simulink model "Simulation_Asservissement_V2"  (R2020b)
settings: Solver=VariableStepAuto  StartTime=0.0  StopTime=12  RelTol=1e-3
libraries: fl_lib x10, nesl_utility x6, ee_lib x1, sdl_lib x1, pid_lib x1

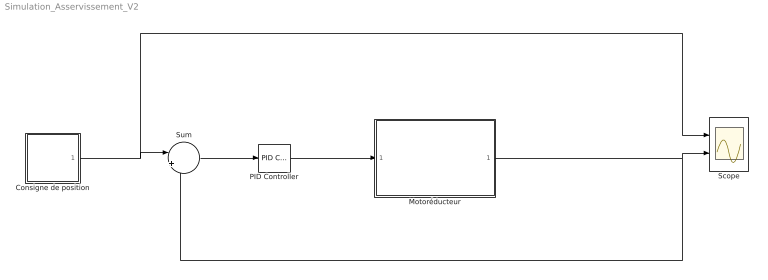
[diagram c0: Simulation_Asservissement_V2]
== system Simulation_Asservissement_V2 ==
  Consigne de position : Subsystem
  Motoréducteur : Subsystem  mask{r_induit=0, k=0.0106, r1=1, Io=0, Rend=100}
      mask prompts: r_induit "Resistance d induit (ohm)"; k "Constante de couple (Nm/A)"; r1 "Rapport de reduction"; Io "Courant a vide (A)"; Rend "Rendement reducteur (%)"
  PID Controller : pid_lib/PID Controller  Controller=PID  Form=Parallel  TimeDomain=Continuous-time  UseExternalTs=off  SampleTime=-1  IntegratorMethod=Forward Euler  FilterMethod=Forward Euler  ControllerParametersSource=internal  P=0.01  I=0  D=0  UseFilter=on  N=150  TunerSelectOption=Transfer Function Based (PID Tuner App)  InitialConditionSource=internal  InitialConditionForIntegrator=0  InitialConditionForFilter=0  DifferentiatorICPrevScaledInput=0  ExternalReset=none  TrackingMode=off  Kt=1  LimitOutput=off  SatLimitsSource=internal  UpperSaturationLimit=inf  LowerSaturationLimit=-inf  LinearizeAsGain=on  AntiWindupMode=none  Kb=1  POutMin=[]  POutMax=[]  IOutMin=[]  IOutMax=[]  DOutMin=[]  DOutMax=[]  NOutMin=[]  NOutMax=[]  SumOutMin=[]  SumOutMax=[]  SaturationOutMin=[]  SaturationOutMax=[]  PParamMin=[]  PParamMax=[]  IParamMin=[]  IParamMax=[]  DParamMin=[]  DParamMax=[]  NParamMin=[]  NParamMax=[]  KbParamMin=[]  KbParamMax=[]  KtParamMin=[]  KtParamMax=[]  KbOutMin=[]  KbOutMax=[]  KtOutMin=[]  KtOutMax=[]  IntegratorOutMin=[]  IntegratorOutMax=[]  FilterOutMin=[]  FilterOutMax=[]  SumI1OutMin=[]  SumI1OutMax=[]  SumI2OutMin=[]  SumI2OutMax=[]  SumI3OutMin=[]  SumI3OutMax=[]  SumI4OutMin=[]  SumI4OutMax=[]  SumDOutMin=[]  SumDOutMax=[]  DifferentiatorOutMin=[]  DifferentiatorOutMax=[]  FilterDiffOutCoefMin=[]  FilterDiffOutCoefMax=[]  ReciprocalOutMin=[]  ReciprocalOutMax=[]  SumDenOutMin=[]  SumDenOutMax=[]  SumNumOutMin=[]  SumNumOutMax=[]  DivideOutMin=[]  DivideOutMax=[]  UdiffTsProdOutMin=[]  UdiffTsProdOutMax=[]  NTsProdOutMin=[]  NTsProdOutMax=[]  UintegralTsProdOutMin=[]  UintegralTsProdOutMax=[]  UngainTsProdOutMin=[]  UngainTsProdOutMax=[]  IntegratorContinuousStateAttributes=''  IntegratorStateMustResolveToSignalObject=off  IntegratorRTWStateStorageClass=Auto  FilterContinuousStateAttributes=''  FilterStateMustResolveToSignalObject=off  FilterRTWStateStorageClass=Auto  ParallelPVariant=InternalParameters  IdealPVariant=Disabled  IVariant=InternalParameters  DVariant=InternalParameters  IntegratorVariant=Continuous  SatVariant=Disabled  AWVariant=Passthrough  PCopyVariant=Disabled  TRVariant=Disabled  FdbkBlocksVariant=Forward  IdealPFdbkVariant=Disabled  SatFdbkVariant=Disabled  DerivativeFilterVariant=ContFilter  NVariant=InternalParameters  NCopyVariant=Disabled  FilterICVariant=InternalICsFilter  IntegratorICVariant=InternalICs  ExternalResetVariant=Disabled  TRSumVariant=Passthrough  SumFdbkVariant=Disabled  SumVariant=Sum_PID  TsampFilterVariant=InternalTs  TsampNgainVariant=Passthrough  TsampIntegralVariant=Passthrough  ExternalSaturationOutDataTypeStr=Inherit: Same as second input
  Scope : Scope  NumInputPorts=2
  Sum : Sum  Inputs=|+-
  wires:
  Sum/1 -> PID Controller/1
  Motoréducteur/1(Out1) -> Scope/2, Sum/2
  PID Controller/1 -> Motoréducteur/1(In1)
  Consigne de position/1(Out1) -> Scope/1, Sum/1

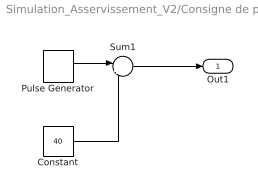
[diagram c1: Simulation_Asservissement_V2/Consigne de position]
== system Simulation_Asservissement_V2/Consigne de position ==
  Constant : Constant  Value=40
  Pulse Generator : DiscretePulseGenerator  PulseType=Time based  Amplitude=40  Period=4  PulseWidth=50
  Sum1 : Sum  Inputs=|++
  Out1 : Outport  VectorParamsAs1DForOutWhenUnconnected=off
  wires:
  Pulse Generator/1 -> Sum1/1
  Sum1/1 -> Out1/1
  Constant/1 -> Sum1/2

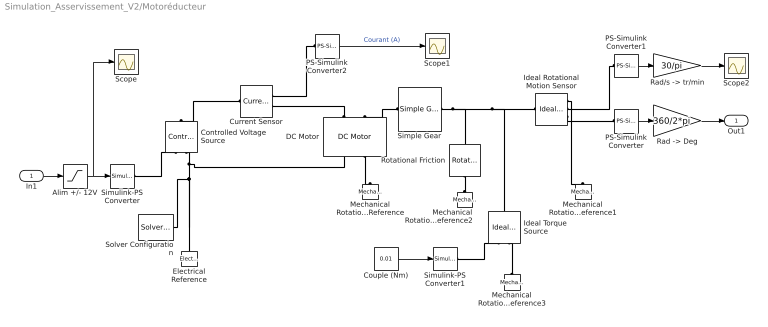
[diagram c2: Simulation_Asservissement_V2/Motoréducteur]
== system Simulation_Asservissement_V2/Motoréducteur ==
  In1 : Inport
  Alim +/- 12V : Saturate  UpperLimit=12  LowerLimit=-12
  Controlled Voltage Source : fl_lib/Electrical/Electrical Sources/Controlled Voltage Source
  Couple (Nm) : Constant  Value=0.01
  Current Sensor : fl_lib/Electrical/Electrical Sensors/Current Sensor
  DC Motor : ee_lib/Electromechanical/Brushed Motors/DC Motor  field_option=ee.enum.field_option.pm  Rf=100 Ohm  Lf=1 H  Laf=0.15 H  If0=0 A  parameterization=1  Ra=r_induit+0.01 Ohm  La=1.2e-2 H  emf_or_torque=2  Kv=k V/(rad/s)  Ki=k N*m/A  T_stall=2.4e-4 N*m  w_max=1.91e+4 rpm  w_rated=1.5e+4 rpm  P_rated=0.08 W  V_rated=1.5 V  J=1e-6 kg*m^2  lam_param=2  lam=0 N*m/(rad/s)  i_noload=Io A  V_i_noload=12 V  speed0=0 rpm  enable_fault_armature=ee.enum.faults.faultEnable.no  rev_faulted=1 / 3  G_faulted_armature=1e-5 S  fault_trigger_armature=ee.enum.faults.faultTrigger.temporal  t_fault_armature=1 s  max_permissible_current_armature=inf A  t_fail_on_current_armature=1 s  enable_fault_field=ee.enum.faults.faultEnable.no  G_faulted_field=1e-5 S  fault_trigger_field=ee.enum.faults.faultTrigger.temporal  t_fault_field=1 s  max_permissible_current_field=inf A  t_fail_on_current_field=1 s  fault_action=ee.enum.faults.faultAction.none  alpha=3.93e-3 1/K  Tmeas=25 degC  thermal_mass=100 J/K  initial_temperature=25 degC
  Electrical Reference : fl_lib/Electrical/Electrical Elements/Electrical Reference
  Ideal Rotational Motion Sensor : fl_lib/Mechanical/Mechanical Sensors/Ideal Rotational Motion Sensor  wrap_angle=simscape.enum.onoff.off  offset=0 rad
  Ideal Torque Source : fl_lib/Mechanical/Mechanical Sources/Ideal Torque Source
  Mechanical Rotational Reference{,1..3} (4 alike) : fl_lib/Mechanical/Rotational Elements/Mechanical Rotational Reference
  PS-Simulink Converter : nesl_utility/PS-Simulink Converter  PhysicalDomain=network_engine_domain  SubClassName=ps_output  LeftPortType=input  RightPortType=output  PseudoPeriodic=off  Frequencies=[]  Unit=1  AffineConversion=off
  PS-Simulink Converter1 : nesl_utility/PS-Simulink Converter  PhysicalDomain=network_engine_domain  SubClassName=ps_output  LeftPortType=input  RightPortType=output  PseudoPeriodic=off  Frequencies=[]  Unit=1  AffineConversion=off
  PS-Simulink Converter2 : nesl_utility/PS-Simulink Converter  PhysicalDomain=network_engine_domain  SubClassName=ps_output  LeftPortType=input  RightPortType=output  PseudoPeriodic=off  Frequencies=[]  Unit=1  AffineConversion=off
  "Rad -> Deg" : Gain  Gain=360/2*pi
  "Rad/s -> tr/min" : Gain  Gain=30/pi
  Rotational Friction : fl_lib/Mechanical/Rotational Elements/Rotational Friction  brkwy_trq=0.01 N*m  brkwy_vel=0.02 rad/s  Col_trq=0.01 N*m  visc_coef=0 N*m/(rad/s)  w_specify=off  w_priority=None  w=0 rad/s  w_nominal_specify=off  w_nominal_unit=rad/s  w_nominal_value=1  t_specify=off  t_priority=None  t=0 N*m  t_nominal_specify=off  t_nominal_unit=N*m  t_nominal_value=1
  Scope : Scope
  Scope1 : Scope
  Scope2 : Scope
  Simple Gear : sdl_lib/Gears/Simple Gear  ratio=1/r1  rotation_direction=3-2*(1)  friction_model=2  mu_visc=[0, 0] N*m/(rad/s)  T_noload=0.1 N*m  T_nom=5 N*m  efficiency_nom=0.8  efficiency=Rend/100  temperature_TLU=[280, 300, 320] K  load_TLU=[1, 5, 10] N*m  efficiency_TLU=[.95, .9, .85]  efficiency_TLU2=[.85, .8, .75; .95, .9, .85; .85, .8, .7]  w_thr=0.01 rad/s  pwr_thr=0.001 W  thermal_mass=50 J/K  enable_faults=simscape.enum.onoff.off  efficiency_fault=0.05  external_fault=simscape.enum.onoff.off  temporal_fault=simscape.enum.onoff.off  fault_time=5 s  fault_angles=pi / 12 rad  report_fault=simscape.enum.assert.action.none  temperature_specify=off  temperature_priority=High  temperature=300 K  temperature_nominal_specify=off  temperature_nominal_unit=K  temperature_nominal_value=1
  Simulink-PS Converter : nesl_utility/Simulink-PS Converter  PhysicalDomain=network_engine_domain  SubClassName=ps_input  LeftPortType=input  RightPortType=output  PseudoPeriodic=off  Frequencies=[]  NoiseDistribution=none  NoiseParameters=[]  Unit=1  AffineConversion=off  FilteringAndDerivatives=provide  SimscapeFilterOrder=1  InputFilterTimeConstant=0.001  UdotUserProvided=0
  Simulink-PS Converter1 : nesl_utility/Simulink-PS Converter  PhysicalDomain=network_engine_domain  SubClassName=ps_input  LeftPortType=input  RightPortType=output  PseudoPeriodic=off  Frequencies=[]  NoiseDistribution=none  NoiseParameters=[]  Unit=1  AffineConversion=off  FilteringAndDerivatives=provide  SimscapeFilterOrder=1  InputFilterTimeConstant=0.001  UdotUserProvided=0
  Solver Configuration : nesl_utility/Solver Configuration  PhysicalDomain=network_engine_domain  SubClassName=solver  LeftPortType=input  RightPortType=generic  Tones=[]  Harmonics=[]  SimulateNoise=off  Profile=off  UseLocalSampling=off  EnableSwitchedLinearOptims=on  FrequencyDomain=off  UseCCode=off  RelTol=0.001  AbsTol=1e-06  MinStep=1e-09  ToWorkspace=off  RevertToSquareIcSolve=off  NumHomotopyIterations=100  PhasorMode=off  PhasorModeNumHarmonics=1  DoDC=off  ResidualTolerance=1e-09  UseLocalSolver=off  LocalSolverChoice=NE_BACKWARD_EULER_ADVANCER  LocalSolverSampleTime=0.001  DoFixedCost=off  MaxNonlinIter=3  MaxModeIter=2  ComputeImpulses=off  ImpulseIterations=2  LinearAlgebra=Sparse  EquationFormulation=NE_TIME_EF  DelaysMemoryBudget=1024  AutomaticFiltering=on  FilteringTimeConstant=0.001  PartitionStorageMethod=AS_NEEDED  PartitionMemoryBudget=1024  PartitionMethod=FAST
  Out1 : Outport  VectorParamsAs1DForOutWhenUnconnected=off
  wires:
  PS-Simulink Converter/1 -> "Rad -> Deg"/1
  Alim +/- 12V/1 -> Scope/1, Simulink-PS Converter/1
  "Rad -> Deg"/1 -> Out1/1
  "Rad/s -> tr/min"/1 -> Scope2/1
  PS-Simulink Converter1/1 -> "Rad/s -> tr/min"/1
  PS-Simulink Converter2/1 -> Scope1/1  "Courant (A)"
  Couple (Nm)/1 -> Simulink-PS Converter1/1
  In1/1 -> Alim +/- 12V/1
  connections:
  DC Motor/LConn1 -- Current Sensor/RConn2
  Simple Gear/RConn1 -- Rotational Friction/LConn1 -- Ideal Torque Source/LConn1 -- Ideal Rotational Motion Sensor/LConn1
  Ideal Rotational Motion Sensor/RConn1 -- Mechanical Rotational Reference1/LConn1
  DC Motor/RConn2 -- Mechanical Rotational Reference/LConn1
  Controlled Voltage Source/RConn2 -- DC Motor/RConn1 -- Electrical Reference/LConn1 -- Solver Configuration/RConn1
  Simple Gear/LConn1 -- DC Motor/LConn2
  Ideal Rotational Motion Sensor/RConn3 -- PS-Simulink Converter/LConn1
  Simulink-PS Converter/RConn1 -- Controlled Voltage Source/RConn1
  PS-Simulink Converter1/LConn1 -- Ideal Rotational Motion Sensor/RConn2
  Current Sensor/LConn1 -- Controlled Voltage Source/LConn1
  PS-Simulink Converter2/LConn1 -- Current Sensor/RConn1
  Rotational Friction/RConn1 -- Mechanical Rotational Reference2/LConn1
  Mechanical Rotational Reference3/LConn1 -- Ideal Torque Source/RConn2
  Simulink-PS Converter1/RConn1 -- Ideal Torque Source/RConn1
